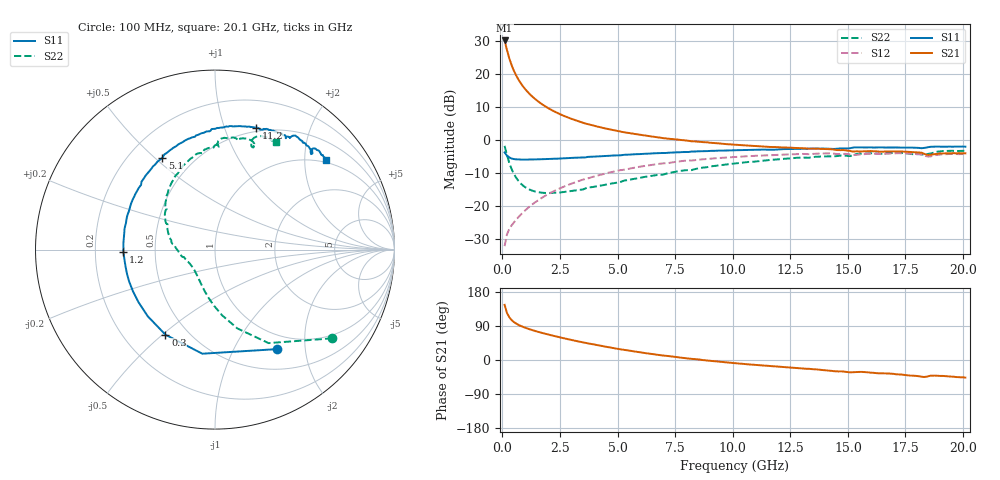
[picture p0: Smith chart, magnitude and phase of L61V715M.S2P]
!  Infineon Technologies AG
! BFR380L3 , PF131585-7, No.6, Th 09.10.01, soldered on pcb-board, measured with PP GSG850
!  Vce=1.75 V,  Ic=15.0 mA
! Common Emitter S-Parameters:  15. November 2001
#  GHz  S  MA  R  50
! f  S11  S21  S12  S22
! GHz  Mag  Ang  Mag  Ang  Mag  Ang  Mag  Ang
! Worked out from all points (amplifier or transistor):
!   201 points, 100 MHz to 20.1 GHz, reference 50 ohm
!   highest |S21| = 30.1 dB at 100 MHz (marker M1)
!   |S21| within 3 dB of that: start of sweep to 207.6 MHz
!   unconditionally stable (mu >= 1): 1.545 GHz to 4.497 GHz
!   at 3.4 GHz: K = 1.02, MAG = 7.9 dB, |S12| = -12.2 dB
!   at 10.1 GHz: K = 0.96, MSG = 1.8 dB, |S12| = -5.1 dB
!   at 20.1 GHz: K = 0.99, MSG = 0.1 dB, |S12| = -4.2 dB
!   S11 on the Smith chart (normalised r, x): 100 MHz: 0.78, -1.50; 300 MHz: 0.38, -0.51; 1.2 GHz: 0.32, -0.01; 5.1 GHz: 0.34, +0.53; 11.2 GHz: 0.46, +1.28; 20.1 GHz: 0.94, +2.54
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0.1  0.6521 -58.3  31.99 145.5  0.02503 66.2  0.8189 -37.1
0.2  0.5843 -96.9  23.15 124.7  0.03752 54.5  0.6004 -60.2
0.3  0.5485 -120.2  17.35 113.1  0.04534 51.3  0.4568 -74.1
0.4  0.5277 -135.2  13.67 105.6  0.05129 51.2  0.3676 -83.9
0.5  0.5173 -145.4  11.21 100.3  0.05696 52.7  0.3099 -91.4
0.6  0.5126 -153.3  9.48 96.3  0.06295 54.1  0.2706 -97.6
0.7  0.5103 -159.5  8.219 92.8  0.06871 55.4  0.2422 -103.1
0.8  0.5087 -164.3  7.24 89.9  0.07489 56.8  0.2214 -107.9
0.9  0.5073 -168.6  6.47 87.4  0.08104 57.7  0.2056 -112.1
1  0.5072 -172.3  5.855 85.0  0.08724 58.6  0.194 -116.1
1.2  0.5106 -178.5  4.917 80.8  0.1003 59.7  0.1781 -123.0
1.6  0.5131 171.4  3.738 73.5  0.127 60.7  0.1627 -134.4
2.1  0.5204 161.7  2.896 65.6  0.1604 59.9  0.1594 -145.3
2.7  0.5331 151.4  2.303 56.9  0.2003 57.7  0.1655 -156.2
3.5  0.5474 139.5  1.828 46.5  0.2533 53.4  0.1796 -166.7
5.1  0.5892 119.9  1.353 28.5  0.351 43.1  0.2317 172.8
6.8  0.6358 102.5  1.095 13.2  0.4383 31.8  0.299 152.8
10.1  0.7025 77.8  0.8521 -8.3  0.5567 10.4  0.444 123.0
11.2  0.7171 71.5  0.8091 -14.0  0.5839 3.5  0.4849 113.9
13.5  0.7408 60.5  0.7439 -24.4  0.6207 -10.0  0.5536 96.7
16.8  0.775 48.2  0.6736 -35.7  0.6256 -25.7  0.6379 76.3
20.1  0.7959 38.7  0.6318 -46.4  0.6187 -39.1  0.6914 60.6
